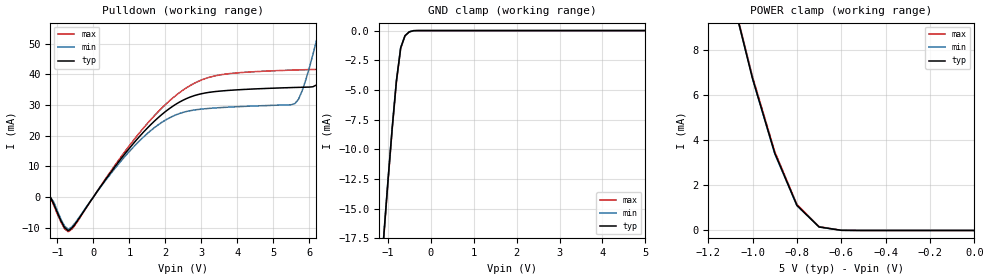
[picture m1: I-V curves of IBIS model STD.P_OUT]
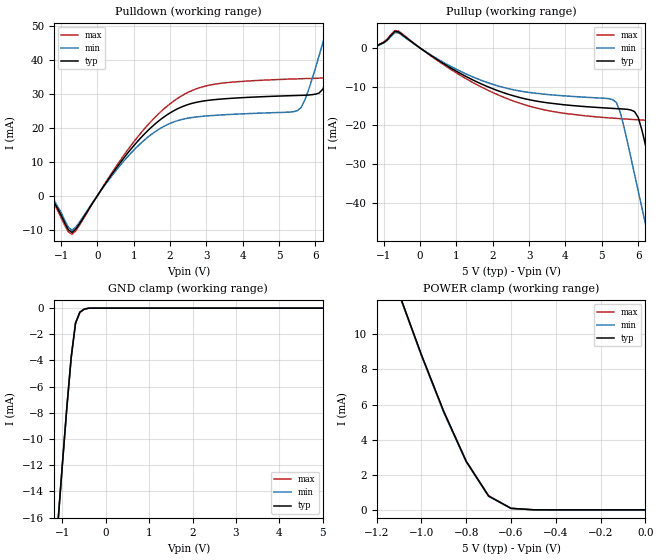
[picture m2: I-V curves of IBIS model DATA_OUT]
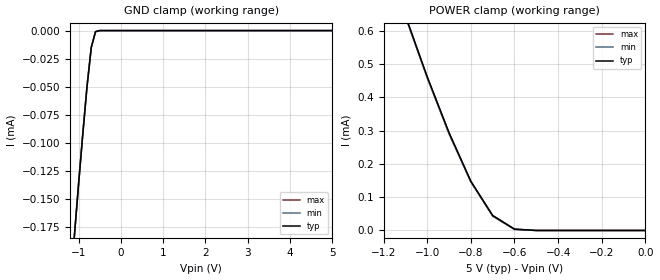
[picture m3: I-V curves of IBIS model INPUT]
| IBIS file rtc72423.ibs
[IBIS ver]   3.2
[File name]   rtc72423.ibs
[File Rev]   1.0
[Date]   Apr. 5, 2007
[Source]   This file orginated at EPSON TOYOCOM Corp
[Copyright]   Copyright EPSON TOYOCOM Corp. 2007
|   Component rtc72423
[Component]   rtc72423
[Manufacturer]   EPSON TOYOCOM
[Package]
| variable   typ   min   max
R_pkg   103m   NA   NA
L_pkg   15nH   NA   NA
C_pkg   573fF   NA   NA
[Pin]  signal_name   model_name   R_pin   L_pin   C_pin
1   STD.P   STD.P_OUT
2   CS0   INPUT
|3   N.C.
4   ALE   INPUT
5   A0   INPUT
|6   N.C.
7   A1   INPUT
|8   N.C.
9   A2   INPUT
10   A3   INPUT
11   READ   INPUT
12   GND   GND
13   WRITE   INPUT
14   D3   DATA_OUT
15   D2   DATA_OUT
16   D1   DATA_OUT
|17   N.C.
|18   N.C.
19   D0   DATA_OUT
20   CS1   INPUT2
|21   N.C.
|22   VDD
|23   VDD
24   VDD   POWER
14T   D3   DATA_IN
15T   D2   DATA_IN
16T   D1   DATA_IN
19T   D0   DATA_IN
| Models and submodels in the file (5): STD.P_OUT (Open_drain), DATA_OUT (Output), INPUT (Input), INPUT2 (Input), DATA_IN (Input)
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|   Model OUTPUT
[Model]   STD.P_OUT
Model_type   Open_drain
Polarity   Non-Inverting
C_comp   1.69pF   1.32pF   1.96pF
[Temperature Range]   25.00   85.00   -40.000
[Voltage Range]   5.0V   4.5V   5.5V
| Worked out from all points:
|   slope of the pulldown table from 0 to 0.75 V, typ, clamps not added: 61.4 ohm
|   GND clamp passes 1 mA (typ) near -0.66 V on its own axis
|   POWER clamp passes 1 mA (typ) near -0.79 V on its own axis
[Pulldown]
| voltage   I(typ)   I(min)   I(max)
-5V       0A         0A         0A
-1.2V     0A         0A         0A
-700mV    -10.99mA   -10.53mA   -11.35mA
1.4V      21.29mA    19.68mA    22.64mA
2.8V      33.08mA    28.39mA    37.1mA
5.6V      35.75mA    30.48mA    41.45mA
5.8V      35.82mA    34.6mA     41.53mA
6.3V      38.39mA    55.67mA    41.68mA
6.8V      58.03mA    80.26mA    42.83mA
7V        67.54mA    90.27mA    48.24mA
8V        116.7mA    140.3mA    93.97mA
10V       215mA      240.4mA    191.2mA
[GND_clamp]
| voltage   I(typ)   I(min)   I(max)
-5V       -196.2mA   -191.2mA   -198.1mA
-1.1V     -17.58mA   -17.5mA    -17.7mA
-1V       -12.83mA   -12.75mA   -12.95mA
-900mV    -8.293mA   -8.221mA   -8.413mA
-800mV    -4.252mA   -4.202mA   -4.353mA
-700mV    -1.45mA    -1.427mA   -1.499mA
-600mV    -433uA     -428uA     -442uA
-500mV    -106uA     -104uA     -109uA
-300mV    0A         0A         0A
5V        0A         0A         0A
[POWER_clamp]
| voltage   I(typ)   I(min)   I(max)
-5V       205.5mA    197.1mA    210mA
-1.1V     10.69mA    10.66mA    10.75mA
-1V       6.733mA    6.729mA    6.822mA
-900mV    3.434mA    3.403mA    3.503mA
-800mV    1.115mA    1.1mA      1.157mA
-700mV    155uA      153uA      171uA
-600mV    7uA        7uA        8uA
0V        0A         0A         0A
[Ramp]
| variable   typ   min   max
dV/dt_r 2.45/8.31n   2.18/8.28n   2.71/8.37n
dV/dt_f 2.45/3.72n   2.16/4.05n   2.76/3.53n
R_load = 300.00
| End [Model] STD.P_OUT
[Model]   DATA_OUT
Model_type   Output
Polarity   Non-Inverting
C_comp   1.69pF   1.32pF   1.96pF
[Temperature Range]   25.00   85.00   -40.000
[Voltage Range]   5.0V   4.5V   5.5V
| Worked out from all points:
|   slope of the pulldown table from 0 to 0.75 V, typ, clamps not added: 65.9 ohm
|   slope of the pullup table from 0 to 0.75 V, typ, clamps not added: 162 ohm
|   GND clamp passes 1 mA (typ) near -0.68 V on its own axis
|   POWER clamp passes 1 mA (typ) near -0.71 V on its own axis
[Pulldown]
| voltage   I(typ)   I(min)   I(max)
-5V       0A         0A         0A
-1.5V     0A         0A         0A
-700mV    -10.81mA   -10.16mA   -11.38mA
1.1V      15.9mA     14.45mA    17.16mA
2.4V      26.43mA    22.59mA    29.84mA
5.5V      29.45mA    24.95mA    34.33mA
5.8V      29.57mA    30.74mA    34.43mA
6.3V      33.47mA    48.62mA    34.6mA
6.8V      50.51mA    67.88mA    36.72mA
7V        58.08mA    75.7mA     42.11mA
8V        96.51mA    114.3mA    78.87mA
10V       172.7mA    191.2mA    154.6mA
[Pullup]
| voltage   I(typ)   I(min)   I(max)
-5V       0A         0A         0A
-1.5V     0A         0A         0A
-600mV    4.205mA    3.955mA    4.429mA
2.3V      -11.56mA   -10.2mA    -12.73mA
5.3V      -15.62mA   -13.36mA   -18.13mA
5.9V      -16.45mA   -32.67mA   -18.51mA
6.3V      -29.23mA   -49.69mA   -18.81mA
6.5V      -37.78mA   -57.99mA   -19.91mA
6.8V      -50.53mA   -70.12mA   -30.15mA
7V        -58.85mA   -77.99mA   -38.63mA
8V        -98.07mA   -116mA     -79.73mA
10V       -174.1mA   -191.8mA   -155.9mA
[GND_clamp]
| voltage   I(typ)   I(min)   I(max)
-5V       -171.2mA   -169.8mA   -170.9mA
-1.1V     -16.19mA   -16.13mA   -16.22mA
-1V       -11.82mA   -11.76mA   -11.86mA
-900mV    -7.606mA   -7.564mA   -7.653mA
-800mV    -3.782mA   -3.743mA   -3.821mA
-700mV    -1.149mA   -1.122mA   -1.169mA
-600mV    -313uA     -306uA     -333uA
-500mV    -78uA      -74uA      -90uA
-300mV    0A         0A         0A
5V        0A         5uA        0A
[POWER_clamp]
| voltage   I(typ)   I(min)   I(max)
-5V       163.9mA    164.8mA    164.2mA
-1.1V     12.34mA    12.29mA    12.33mA
-1V       8.837mA    8.791mA    8.84mA
-900mV    5.599mA    5.538mA    5.612mA
-800mV    2.766mA    2.739mA    2.785mA
-700mV    786uA      772uA      810uA
-600mV    86uA       83uA       88uA
-500mV    5uA        5uA        5uA
0V        0A         0A         0A
[Ramp]
| variable   typ   min   max
dV/dt_r 1.85/18.08n   1.58/18.47n   2.09/17.76n
dV/dt_f 2.45/15.24n   2.16/15.75n   2.71/14.88n
R_load = 300.00
| End [Model] DATA_OUT
|   Model INPUT
[Model]   INPUT
Model_type   Input
Polarity   Non-Inverting
Vinl =   0.8V
Vinh =   2.2V
C_comp   0.80pF   0.60pF   1.00pF
[Temperature Range]   25.00   85.00   -40.00
[Voltage Range]   5.0V   4.5V   5.50V
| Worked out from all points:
|   GND clamp passes 1 mA (typ) near -2.77 V on its own axis
|   POWER clamp passes 1 mA (typ) near -1.28 V on its own axis
[GND_clamp]
| voltage   I(typ)   I(min)   I(max)
-5V       -2.114mA   -2.114mA   -2.114mA
-1.1V     -183uA     -183uA     -183uA
-1V       -137uA     -136uA     -136uA
-900mV    -92uA      -91uA      -92uA
-800mV    -50uA      -49uA      -49uA
-700mV    -15uA      -15uA      -15uA
-600mV    -1uA       -1uA       -1uA
-500mV    0A         0A         0A
5V        0A         0A         0A
[POWER_clamp]
| voltage   I(typ)   I(min)   I(max)
-5V       8.995mA    8.999mA    9mA
-1.1V     646uA      643uA      645uA
-1V       462uA      459uA      461uA
-900mV    294uA      290uA      293uA
-800mV    148uA      146uA      147uA
-700mV    45uA       43uA       45uA
-600mV    4uA        3uA        4uA
-500mV    0A         0A         0A
0V        0A         0A         0A
